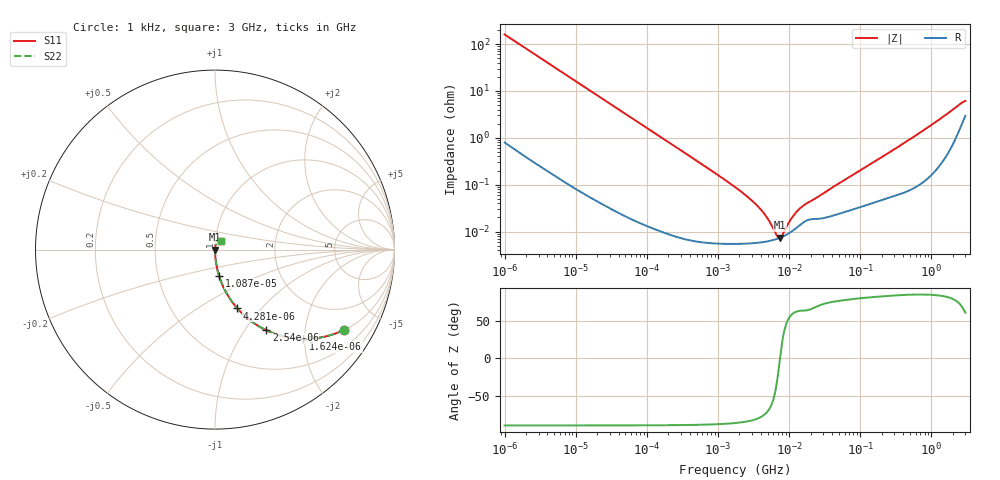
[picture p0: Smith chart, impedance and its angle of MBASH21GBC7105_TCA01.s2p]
! MBASH21GBC7105_TCA01  S-PARAMETER MODEL  ( Standard Model )
! Model Generated by TAIYO YUDEN Corporation (http://www.ty-top.com)
! Version 1.0
! TAIYO YUDEN Control No. 220601
! Copyright(c) 2016 TAIYO YUDEN CO.,LTD. All Rights Reserved.
! Product Description (link to TY-COMPAS)
! https://ds.yuden.co.jp/TYCOMPAS/or/detail?pn=MBASH21GBC7105KTCA01&u=M
! Products Name : Multilayer Ceramic Capacitors
! Characteristics :
!  Capacitance : 1 [uF] , Rated Voltage : 100 [V] , TCC : X7S
!  Case Size : 2.0 x 1.25 / 0.079 x 0.049 [mm/inch] , Thickness : 1.25 / 0.049 [mm/inch]
!  (Conditions: Temperature = 25 [degC] , DC Bias Voltage = 0 [V])
! External Node Assignments :
!  1  o---| |---o  2
! GND o---------o GND
! Frequency Range : 1kHz  -  3GHz  [ 401 STEP ]
# MHZ S RI R 50
! Freq[MHz].  S11 Real  S11 Imag  S21 Real  S21 Imag  S12 Real  S12 Imag  S22 Real  S22 Imag
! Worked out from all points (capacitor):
!   401 points, 1 kHz to 3 GHz, reference 50 ohm
!   read as one part in series: C = 995 nF near 1.077 kHz
!   lowest |Z| = 7.36 mohm at 7.414 MHz (marker M1)
!   series resonance near 7.422 MHz, so ESL is about 460 pH
!   S11 on the Smith chart (normalised r, x): 1 kHz: 1.02, -3.19; 1.624 kHz: 1.01, -1.97; 2.54 kHz: 1.01, -1.26; 4.281 kHz: 1.00, -0.75; 10.87 kHz: 1.00, -0.30; 3 GHz: 1.06, +0.11
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0.001  0.7174 -0.4478  0.2826 0.4478  0.2826 0.4478  0.7174 -0.4478
0.001624  0.4925 -0.4975  0.5075 0.4975  0.5075 0.4975  0.4925 -0.4975
0.00254  0.2854 -0.4492  0.7146 0.4492  0.7146 0.4492  0.2854 -0.4492
0.004281  0.1243 -0.3275  0.8757 0.3275  0.8757 0.3275  0.1243 -0.3275
0.010873  0.0221 -0.1446  0.9779 0.1446  0.9779 0.1446  0.0221 -0.1446
0.01216  0.0179 -0.1299  0.9821 0.1299  0.9821 0.1299  0.0179 -0.1299
0.033275  0.00263 -0.0484  0.9974 0.0484  0.9974 0.0484  0.00263 -0.0484
0.147855  0.000224 -0.011  0.9998 0.011  0.9998 0.011  0.000224 -0.011
1.732051  5.53e-05 -0.000889  0.9999 0.000889  0.9999 0.000889  5.53e-05 -0.000889
2.709407  5.59e-05 -0.00052  0.9999 0.00052  0.9999 0.00052  5.59e-05 -0.00052
3.789741  5.81e-05 -0.000317  0.9999 0.000317  0.9999 0.000317  5.81e-05 -0.000317
4.739869  6.1e-05 -0.000203  0.9999 0.000203  0.9999 0.000203  6.1e-05 -0.000203
6.387174  6.8e-05 -6.56e-05  0.9999 6.56e-05  0.9999 6.56e-05  6.8e-05 -6.56e-05
7.414467  7.36e-05 -4.3e-07  0.9999 4.3e-07  0.9999 4.3e-07  7.36e-05 -4.3e-07
8.606987  8.14e-05 6.42e-05  0.9999 -6.42e-05  0.9999 -6.42e-05  8.14e-05 6.42e-05
11.1738  0.000104 0.000178  0.9999 -0.000178  0.9999 -0.000178  0.000104 0.000178
13.97519  0.000136 0.000274  0.9999 -0.000274  0.9999 -0.000274  0.000136 0.000274
21.06097  0.000184 0.000425  0.9998 -0.000425  0.9998 -0.000425  0.000184 0.000425
256.0921  0.000551 0.00485  0.9994 -0.00485  0.9994 -0.00485  0.000551 0.00485
944.3747  0.00178 0.0176  0.9982 -0.0176  0.9982 -0.0176  0.00178 0.0176
2584.342  0.0195 0.0491  0.9805 -0.0491  0.9805 -0.0491  0.0195 0.0491
3000  0.0312 0.0503  0.9688 -0.0503  0.9688 -0.0503  0.0312 0.0503
